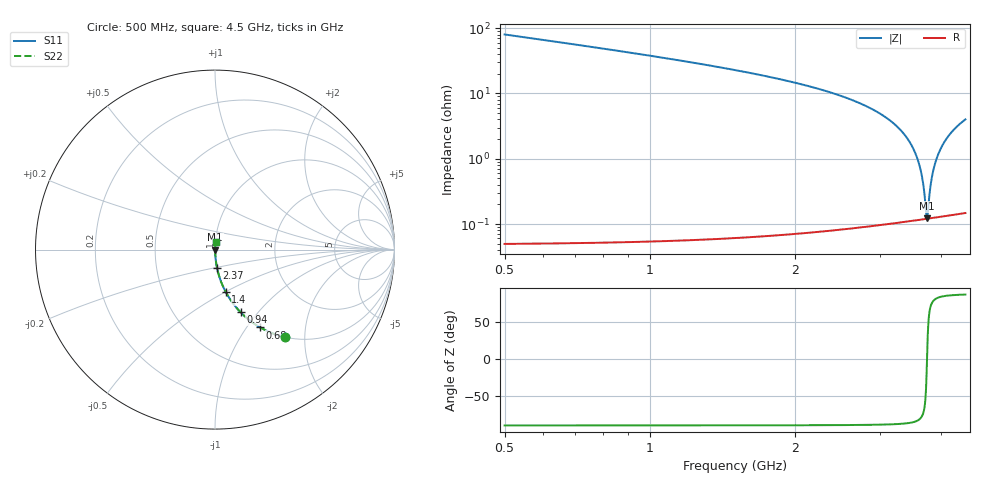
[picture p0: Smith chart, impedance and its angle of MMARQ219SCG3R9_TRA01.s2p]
! MMARQ219SCG3R9_TRA01  S-PARAMETER MODEL  ( General Type )
! Model Generated by TAIYO YUDEN Corporation (http://www.ty-top.com)
! Version 1.0
! TAIYO YUDEN Control No. 180601
! Copyright(c) 2018 TAIYO YUDEN CO.,LTD. All Rights Reserved.
! Product Description (link to TY-COMPAS)
! https://ds.yuden.co.jp/TYCOMPAS/or/detail?pn=MMARQ219SCG3R9BTRA01&u=M
! Products Name : Multilayer Ceramic Capacitors
! Characteristics :
!  Capacitance : 3.9 pF , Rated Voltage : 250V , TCC : CG / C0G
!  Case Size : 2.0 x 1.25 / 0.079 x 0.049 [mm/inch] , Thickness : 0.85 / 0.033 [mm/inch]
!  (Conditions: Temperature = 25 degC , DC Bias Current/Voltage = 0A / 0V)
! External Node Assignments :
!  1  o---| |---o  2
! GND o---------o GND
! Frequency Range : 500MHz  -  4500MHz  [ 401 STEP ]
# MHz S RI R 50
! Freq[MHz].  S11 Real  S11 Imag  S21 Real  S21 Imag  S12 Real  S12 Imag  S22 Real  S22 Imag
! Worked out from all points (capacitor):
!   401 points, 500 MHz to 4.5 GHz, reference 50 ohm
!   read as one part in series: C = 3.9 pF near 520 MHz
!   lowest |Z| = 121 mohm at 3.75 GHz (marker M1)
!   series resonance near 3.747 GHz, so ESL is about 460 pH
!   S11 on the Smith chart (normalised r, x): 500 MHz: 1.00, -1.60; 680 MHz: 1.00, -1.16; 940 MHz: 1.00, -0.81; 1.4 GHz: 1.00, -0.50; 2.37 GHz: 1.00, -0.21; 4.5 GHz: 1.00, +0.08
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500  0.3915 -0.4878  0.6085 0.4878  0.6085 0.4878  0.3915 -0.4878
680  0.2523 -0.4339  0.7477 0.4339  0.7477 0.4339  0.2523 -0.4339
940  0.1424 -0.3488  0.8576 0.3488  0.8576 0.3488  0.1424 -0.3488
1170  0.0906 -0.2862  0.9094 0.2862  0.9094 0.2862  0.0906 -0.2862
1400  0.0597 -0.2357  0.9403 0.2357  0.9403 0.2357  0.0597 -0.2357
1840  0.0282 -0.1634  0.9718 0.1634  0.9718 0.1634  0.0282 -0.1634
2370  0.0113 -0.102  0.9887 0.102  0.9887 0.102  0.0113 -0.102
2500  0.00893 -0.0896  0.9911 0.0896  0.9911 0.0896  0.00893 -0.0896
3170  0.00235 -0.0364  0.9977 0.0364  0.9977 0.0364  0.00235 -0.0364
3400  0.00153 -0.0211  0.9985 0.0211  0.9985 0.0211  0.00153 -0.0211
3560  0.00126 -0.0111  0.9987 0.0111  0.9987 0.0111  0.00126 -0.0111
3660  0.0012 -0.00511  0.9988 0.00511  0.9988 0.00511  0.0012 -0.00511
3690  0.00119 -0.00334  0.9988 0.00334  0.9988 0.00334  0.00119 -0.00334
3730  0.0012 -0.001  0.9988 0.001  0.9988 0.001  0.0012 -0.001
3750  0.0012 0.000157  0.9988 -0.000157  0.9988 -0.000157  0.0012 0.000157
3760  0.00121 0.000734  0.9988 -0.000734  0.9988 -0.000734  0.00121 0.000734
3800  0.00123 0.00303  0.9988 -0.00303  0.9988 -0.00303  0.00123 0.00303
3840  0.00126 0.0053  0.9987 -0.0053  0.9987 -0.0053  0.00126 0.0053
3930  0.00137 0.0103  0.9986 -0.0103  0.9986 -0.0103  0.00137 0.0103
4060  0.00161 0.0174  0.9984 -0.0174  0.9984 -0.0174  0.00161 0.0174
4250  0.00213 0.0273  0.9979 -0.0273  0.9979 -0.0273  0.00213 0.0273
4500  0.00306 0.0398  0.9969 -0.0398  0.9969 -0.0398  0.00306 0.0398
